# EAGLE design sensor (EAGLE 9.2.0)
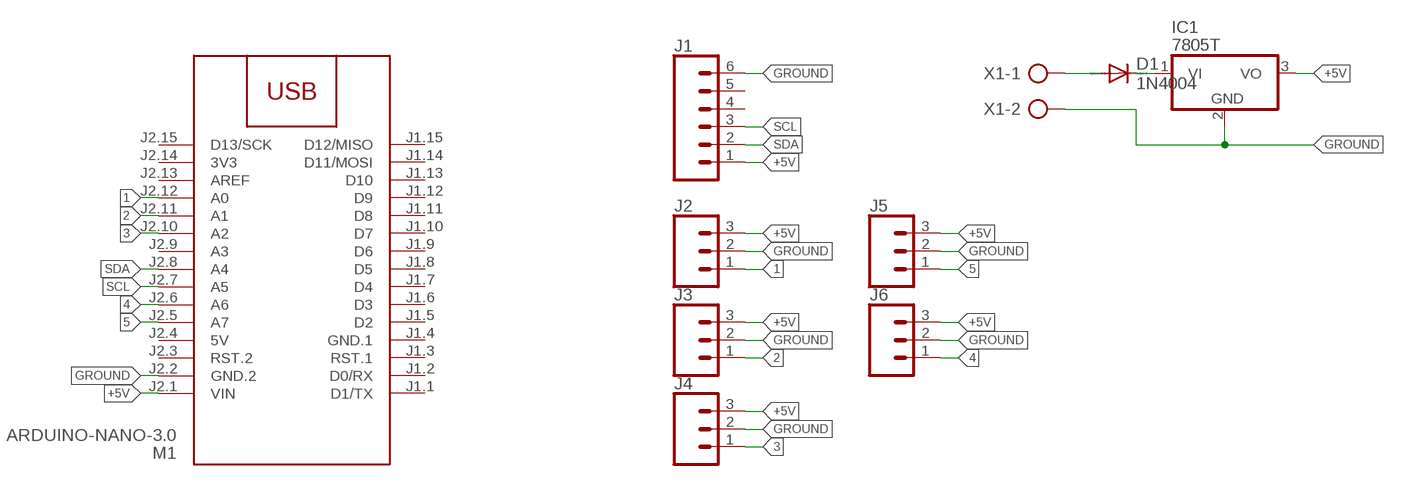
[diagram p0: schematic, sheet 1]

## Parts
D1  1N4004  [DO41-10]
IC1  7805T  [TO220H]
J1  CONN_06LONGPADS  [1X06_LONGPADS]
J2  CONN_03LONGPADS  [1X03_LONGPADS]
J3  CONN_03LONGPADS  [1X03_LONGPADS]
J4  CONN_03LONGPADS  [1X03_LONGPADS]
J5  CONN_03LONGPADS  [1X03_LONGPADS]
J6  CONN_03LONGPADS  [1X03_LONGPADS]
M1  ARDUINO-NANO-3.0  [ARDUINO-NANO-3.0]
X1  AK300/2  [AK300/2]

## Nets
1: J2.1 M1.J2.12(A0)
2: J3.1 M1.J2.11(A1)
3: J4.1 M1.J2.10(A2)
4: J6.1 M1.J2.6(A6)
5: J5.1 M1.J2.5(A7)
+5V: IC1.3(VO) J1.1 J2.3 J3.3 J4.3 J5.3 J6.3 M1.J2.1(VIN)
GROUND: IC1.2(GND) J1.6 J2.2 J3.2 J4.2 J5.2 J6.2 M1.J2.2(GND.2) X1.2
N$1: D1.A X1.1
N$4: D1.C IC1.1(VI)
SCL: J1.3 M1.J2.7(A5)
SDA: J1.2 M1.J2.8(A4)
Unconnected: J1.4 J1.5 M1.J1.1(D1/TX) M1.J1.2(D0/RX) M1.J1.3(RST.1) M1.J1.5(D2) M1.J1.6(D3) M1.J1.7(D4) M1.J1.8(D5) M1.J1.9(D6) M1.J1.10(D7) M1.J1.11(D8) M1.J1.12(D9) M1.J1.13(D10) M1.J1.14(D11/MOSI) M1.J1.15(D12/MISO) M1.J2.3(RST.2) M1.J2.9(A3) M1.J2.13(AREF) M1.J2.15(D13/SCK)

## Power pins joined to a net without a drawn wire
3V3: M1.J2.14(3V3)
5V: M1.J2.4(5V)
GND.1: M1.J1.4(GND.1)

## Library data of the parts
D1 = diode:1N4004: DIODE
IC1 = linear:78*: Positive VOLTAGE REGULATOR Source: http://cache.national.com/ds/LM/LM78L05.pdf http://www.fairchildsemi.com/ds/LM/LM7805.pdf
J1 = SparkFun-Connectors:CONN_06: Multi connection point. Often used as Generic Header-pin footprint for 0.1 inch spaced/style header connections On any of the 0.1 inch spaced packages, you can populate with these: Break Away Headers - Straight (PRT-00116) Break Away Male Headers - Right Angle (PRT-00553) Female Headers (PRT-00115)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
J2-J6 = SparkFun-Connectors:CONN_03: Multi connection point. Often used as Generic Header-pin footprint for 0.1 inch spaced/style header connections On any of the 0.1 inch spaced packages, you can populate with these: Break Away Headers - Straight (PRT-00116) Break Away Male Headers - Right Angle (PRT-00553) Female Headers (PRT-00115)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
M1 = diy-modules:ARDUINO-NANO-3.0: Arduino Nano 3.0 and compatible devices More details available here: https://www.arduino.cc/en/Main/ArduinoBoardNano Click here to find device on ebay.com
X1 = con-ptr500:AK300/2: CONNECTOR; OC_FARNELL: unknown; OC_NEWARK: unknown

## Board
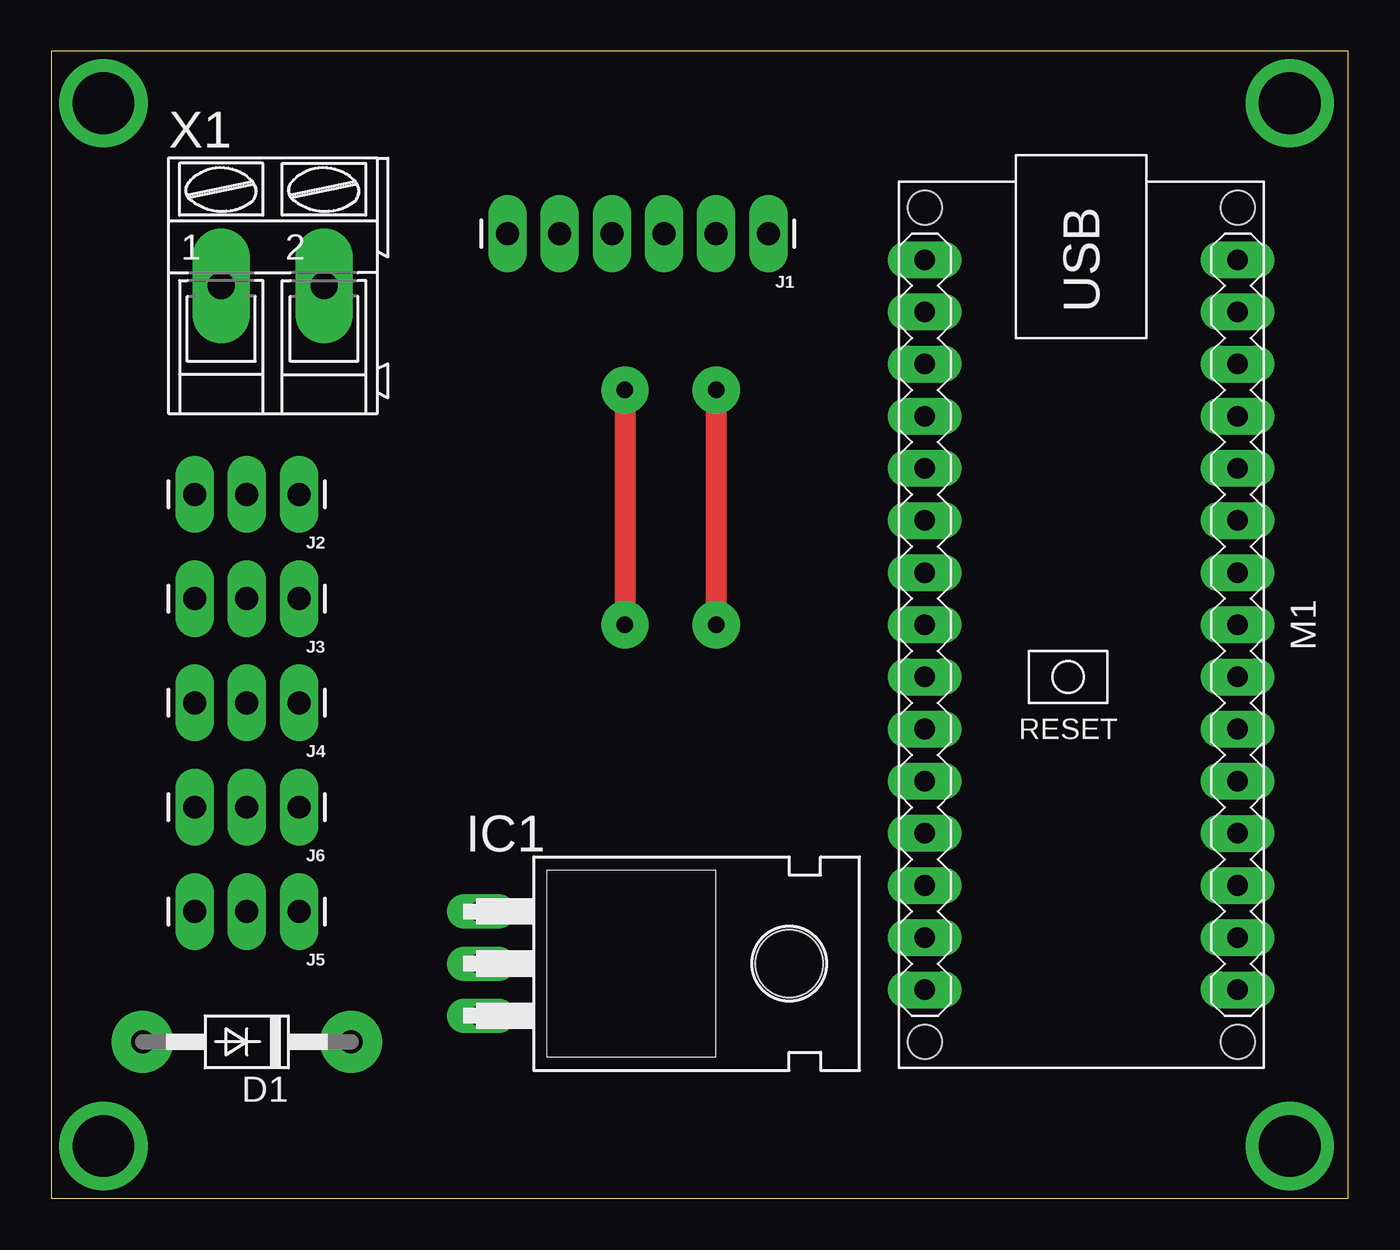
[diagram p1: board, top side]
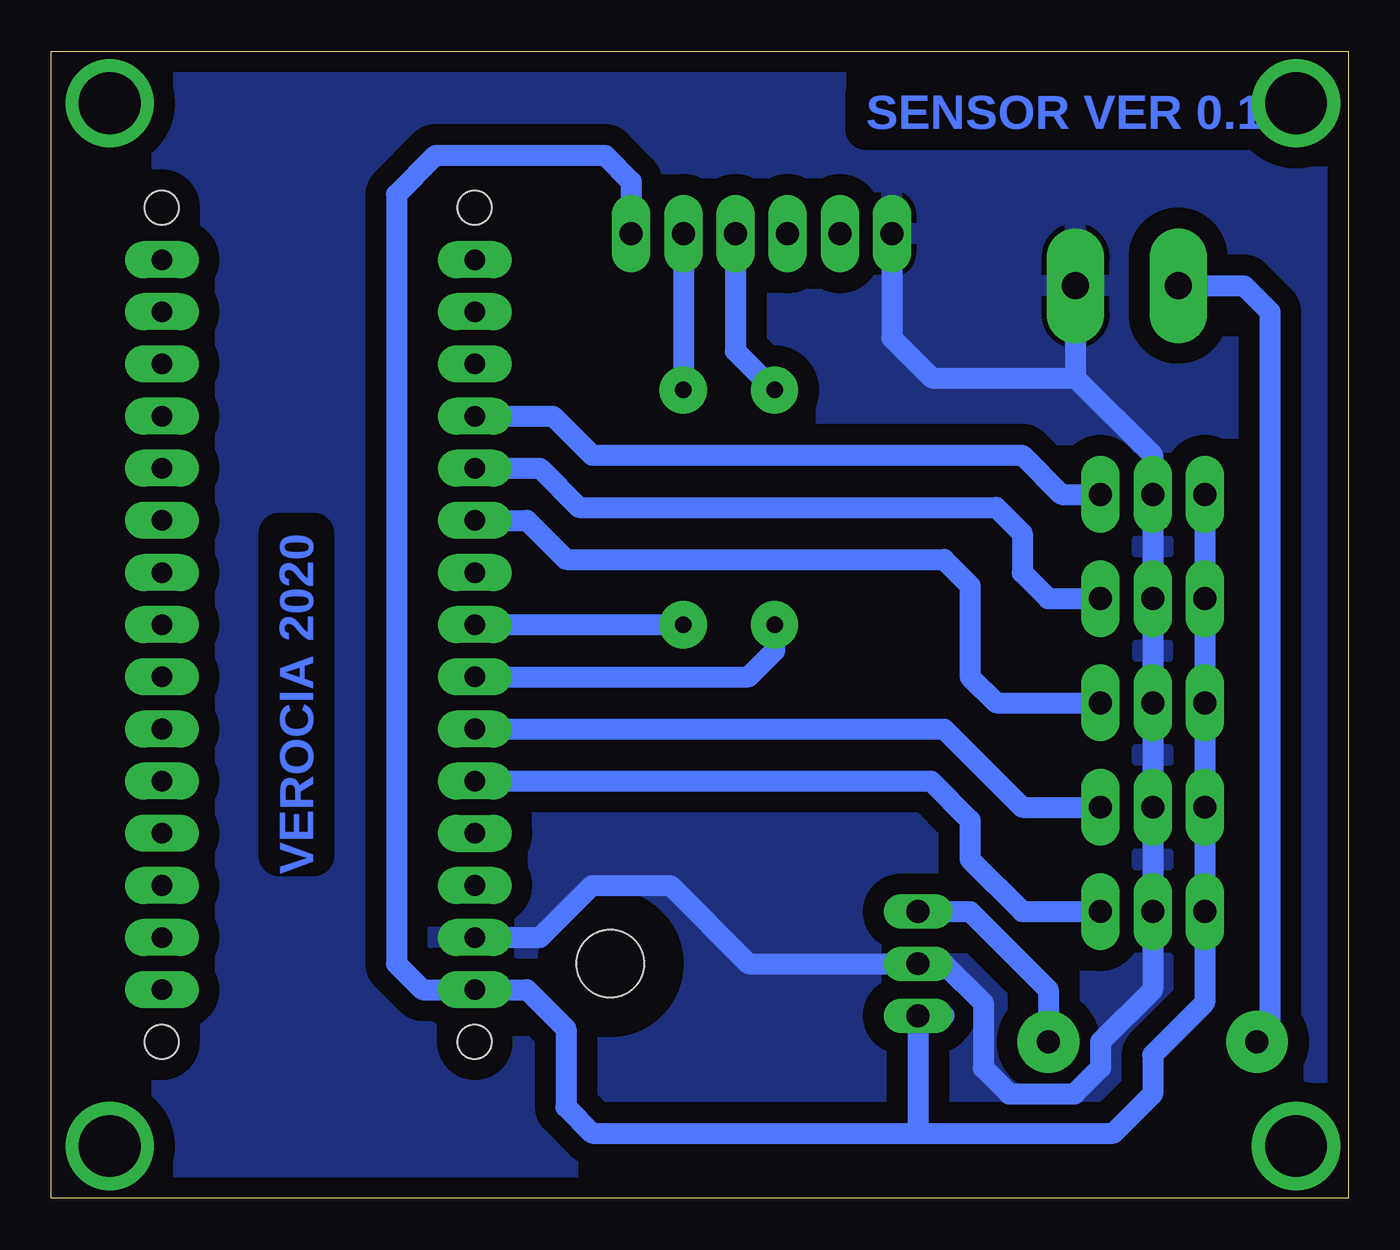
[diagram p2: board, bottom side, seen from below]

Size 63.17 x 55.87 mm. Coordinates in mm from the lower left corner, seen from the top.
Outline: 0,0 63.17,0 63.17,55.87 0,55.87 0,0
Copper layers (1*16): Top 0.035mm / dielectric 1.5mm / Bottom 0.035mm
Design rules "default": minimum track width 6mil, minimum drill 0.35mm, track to track 6mil, track to pad 6mil, pad to pad 6mil, via to via 6mil, smd to smd 6mil, copper to edge 40mil, drill to drill 6mil, minimum pad ring 10mil, minimum via ring 8mil, stop-mask expansion 4mil, vias tented up to drill 0mil, thermal gap 10mil

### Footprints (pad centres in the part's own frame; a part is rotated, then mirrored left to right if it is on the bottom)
DO41-10 = drill 1.118 pad 3: A 5.08,0; C -5.08,0
TO220H = drill 1.118 long: 1 -2.54,-10.16; 2 0,-10.16; 3 2.54,-10.16 | hole 3.302: 0,4.826
1X06_LONGPADS = drill 1.118 pad 1.88 long: 1 0,0; 2 2.54,0; 3 5.08,0; 4 7.62,0; 5 10.16,0; 6 12.7,0
1X03_LONGPADS = drill 1.118 pad 1.88 long: 1 0,0; 2 2.54,0; 3 5.08,0
ARDUINO-NANO-3.0 = drill 1 pad 1.8 long: J1.1 17.78,7.62; J1.2 15.24,7.62; J1.3 12.7,7.62; J1.4 10.16,7.62; J1.5 7.62,7.62; J1.6 5.08,7.62; J1.7 2.54,7.62; J1.8 0,7.62; J1.9 -2.54,7.62; J1.10 -5.08,7.62; J1.11 -7.62,7.62; J1.12 -10.16,7.62; J1.13 -12.7,7.62; J1.14 -15.24,7.62; J1.15 -17.78,7.62; J2.1 17.78,-7.62; J2.2 15.24,-7.62; J2.3 12.7,-7.62; J2.4 10.16,-7.62; J2.5 7.62,-7.62; J2.6 5.08,-7.62; J2.7 2.54,-7.62; J2.8 0,-7.62; J2.9 -2.54,-7.62; J2.10 -5.08,-7.62; J2.11 -7.62,-7.62; J2.12 -10.16,-7.62; J2.13 -12.7,-7.62; J2.14 -15.24,-7.62; J2.15 -17.78,-7.62 | hole 1.651: -20.32,7.62; -20.32,-7.62; 20.32,-7.62; 20.32,7.62
AK300/2 = drill 1.321 pad 2.8 long: 1 -2.515,0; 2 2.489,0

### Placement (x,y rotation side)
D1  9.53,7.62 180 top
IC1  31.11,11.43 270 top
J1  34.92,46.99 180 top
J2  12.06,34.29 180 top
J3  12.06,29.21 180 top
J4  12.06,24.13 180 top
J5  12.06,13.97 180 top
J6  12.06,19.05 180 top
M1  50.16,27.94 270 top
X1  10.79,44.45 0 top

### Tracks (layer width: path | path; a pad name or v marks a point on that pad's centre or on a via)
1
  Bottom 1.016: J2.1 13.97,34.29 15.88,36.2 36.83,36.2 38.73,38.1 M1.J2.12
2
  Bottom 1.016: M1.J2.11 39.37,35.56 37.47,33.66 17.14,33.66 15.88,32.39 15.88,30.48 14.61,29.21 J3.1
3
  Bottom 1.016: M1.J2.10 40.01,33.02 38.1,31.11 19.68,31.11 18.41,29.84 18.41,25.4 17.14,24.13 J4.1
4
  Bottom 1.016: J6.1 15.88,19.05 19.68,22.86 M1.J2.6
5
  Bottom 1.016: J5.1 15.88,13.97 18.41,16.51 18.41,18.41 20.32,20.32 M1.J2.5 43.18,20.32
+5V
  Bottom 1.016: J2.3 J3.3 J4.3 J6.3 J5.3 6.99,9.53 9.53,6.99 9.53,5.08 11.43,3.17 20.95,3.17 | 19.68,8.89 IC1.3 20.95,3.17 | 20.95,3.17 36.83,3.17 38.1,4.45 38.1,8.26 40.01,10.16 M1.J2.1 45.09,10.16 46.35,11.43 46.35,48.9 44.45,50.8 36.2,50.8 34.92,49.53 J1.1
GROUND
  Bottom 1.016: X1.2 13.28,39.95 | 13.28,39.95 9.53,36.2 J2.2 J3.2 J4.2 J6.2 J5.2 9.53,10.16 12.06,7.62 12.06,6.35 13.34,5.08 16.51,5.08 17.78,6.35 17.78,9.53 19.68,11.43 IC1.2 29.21,11.43 33.02,15.24 36.83,15.24 39.37,12.7 M1.J2.2 43.18,12.7 | J1.6 22.23,41.91 20.27,39.95 13.28,39.95
  pour Bottom (isolate 1.016): 0,55.88 63.5,55.88 63.5,0 0,0
N$1
  Bottom 1.016: D1.A 3.81,8.26 3.81,43.18 5.08,44.45 X1.1
N$2  (via drill 3 pad 4.3)
  other vias: 2.54,53.34
N$3  (via drill 3 pad 4.3)
  other vias: 60.33,53.34
N$4
  Bottom 1.016: D1.C 14.61,10.16 18.41,13.97 IC1.1
N$5  (via drill 3 pad 4.3)
  other vias: 60.33,2.54
N$6  (via drill 3 pad 4.3)
  other vias: 2.54,2.54
SCL  (via drill 0.8 pad 2.3)
  Top 1.016: v27.94,39.37 v27.94,27.94
  Bottom 1.016: J1.3 29.84,41.27 v27.94,39.37 | v27.94,27.94 27.94,26.67 29.21,25.4 M1.J2.7
SDA  (via drill 0.8 pad 2.3)
  Top 1.016: v32.38,39.37 v32.38,27.94
  Bottom 1.016: J1.2 v32.38,39.37 | M1.J2.8 v32.38,27.94

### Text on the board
Bottom: SENSOR VER 0.1 | VEROCIA 2020

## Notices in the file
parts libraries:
diy-modules: Released under the Creative Commons Attribution 4.0 International License: http://creativecommons.org/licenses/by/4.0
SparkFun-Connectors: Licensing: Creative Commons ShareAlike 4.0 International - https://creativecommons.org/licenses/by-sa/4.0
